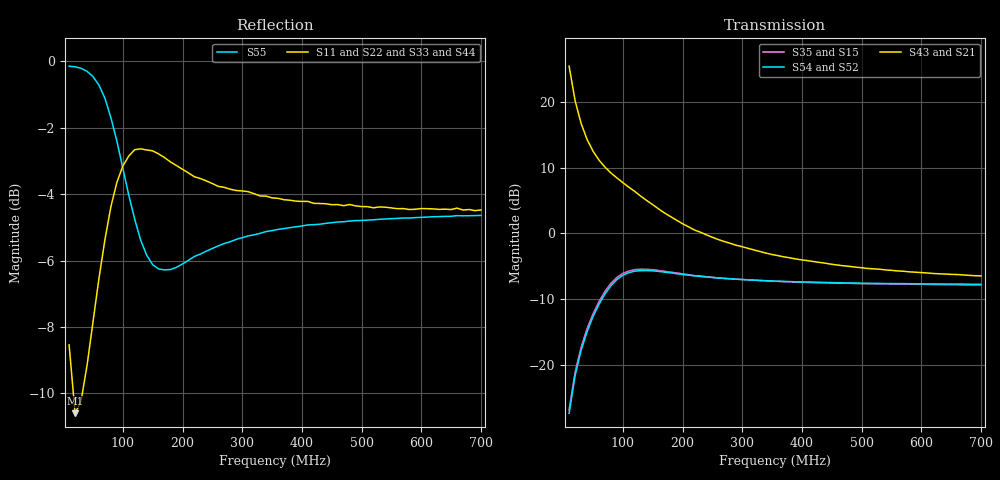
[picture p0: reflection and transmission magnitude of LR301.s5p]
!  POLYFET RF DEVICES
!  LR301 (Each Side)
!  S PARAMETERS
!  VDS=28V, IDQ=400mA
! Date: Wed Mar 05 14:34:01 2003
!AWR Design Environment (2053) Wed Feb 04 15:26:32 2004
!freq-unit  param-type  data-format  keyword  impedance-ohms
# MHz  S  MA  R  50
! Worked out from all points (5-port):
!   70 points, 10 MHz to 700 MHz, reference 50 ohm
!   strongest paths, dB at 10 MHz, 180 MHz, 360 MHz, 530 MHz, 700 MHz:
!     S43: 25.4, 2.6, -3.4, -5.4, -6.4
!     S21: 25.4, 2.6, -3.4, -5.4, -6.4
!     S54: -27.3, -6.0, -7.3, -7.6, -7.7
!     S52: -27.3, -6.0, -7.3, -7.6, -7.7
!     S35: -26.8, -5.9, -7.3, -7.6, -7.8
!     S15: -26.8, -5.9, -7.3, -7.6, -7.8
!   lowest |S11| = -10.6 dB at 20 MHz (marker M1), VSWR 1.84, Z = 54.1 - j31.9 ohm
!   |S11| at or under -10 dB: 17.1 MHz to 32.15 MHz (15.05 MHz wide, 61.1 % of centre)
